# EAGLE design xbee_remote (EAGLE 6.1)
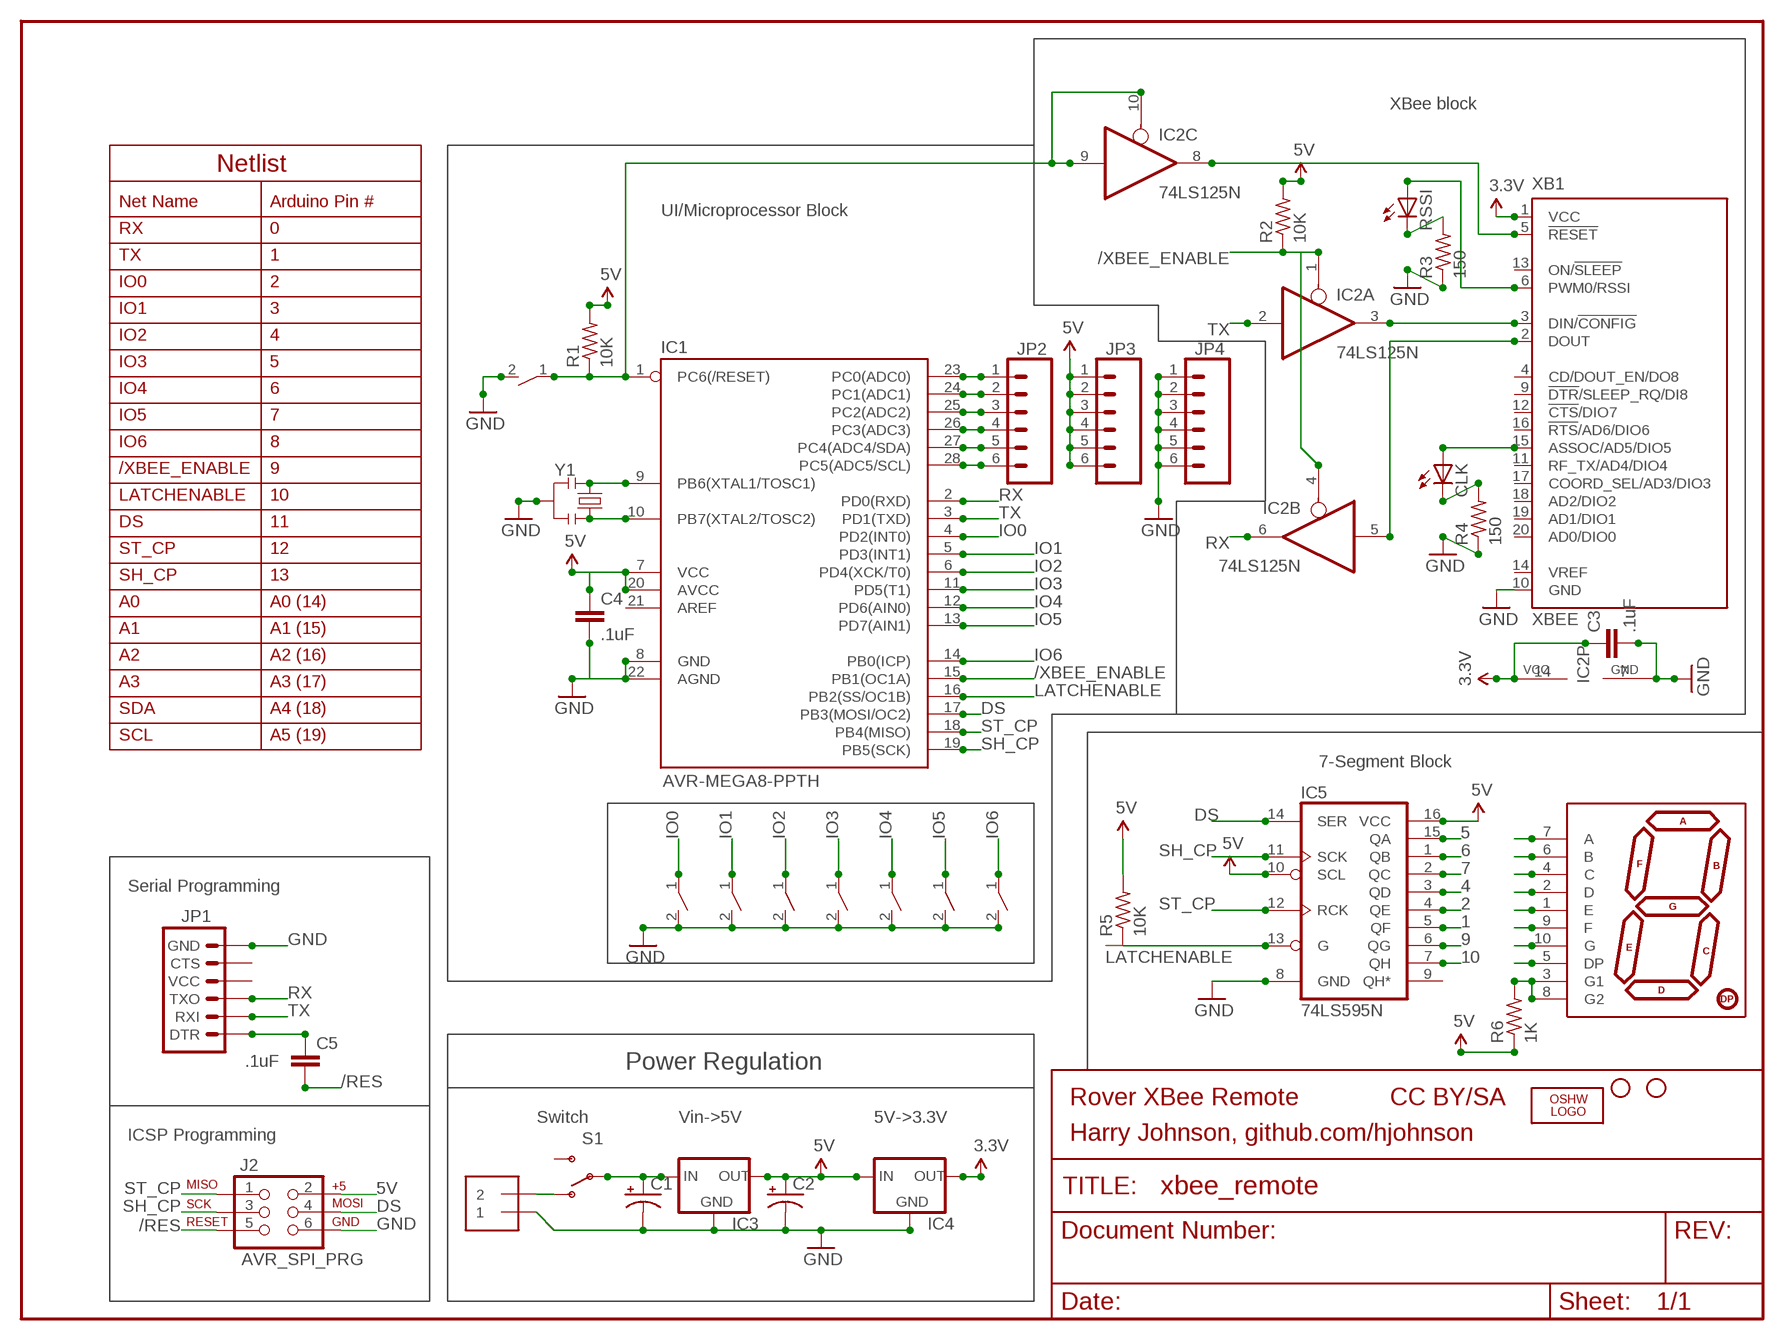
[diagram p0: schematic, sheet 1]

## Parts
C1  CAP_POLPTH1  [CPOL-RADIAL-100UF-25V]
C2  CAP_POLPTH2  [CPOL-RADIAL-10UF-25V]
C3  .1uF  CAPPTH2  [CAP-PTH-SMALL2]
C4  .1uF  CAPPTH2  [CAP-PTH-SMALL2]
C5  .1uF  CAPPTH2  [CAP-PTH-SMALL2]
CLK  LED3MM  [LED3MM]
IC1  AVR-MEGA8-PPTH  [DIL28-3]
IC2  74LS125N  [DIL14]
IC3  V_REG_78XXSIDE  [78XXL]
IC4  MCP1700TRI  [TO92]
IC5  74LS595N  [DIL16]
J1  1X2-3.5MM  [3.5MMTERM]
J2  AVR_SPI_PRG  AVR_SPI_PRG_6PTH  [2X3]
JP1  ARDUINO_SERIAL_PROGRAMPTH  [1X06]
JP2  M06SIP  [1X06]
JP3  M06SIP  [1X06]
JP4  M06SIP  [1X06]
JP5  STAND-OFF  [STAND-OFF]
JP6  STAND-OFF  [STAND-OFF]
LOGO1  OSHW_LOGO_FILLX0150-NT  [OSHW_FILLX150_NOTEXT]
R1  10K  R-US_0207/10  [0207/10]
R2  10K  R-US_0207/10  [0207/10]
R3  150  R-US_0207/10  [0207/10]
R4  150  R-US_0207/10  [0207/10]
R5  10K  R-US_0207/10  [0207/10]
R6  1K  R-US_0207/10  [0207/10]
RSSI  LED3MM  [LED3MM]
S1  SWITCH-SPSTPTH  [SWITCH-SPDT]
U$4  7-SEGMENT-DISPLAY-1"-RED  [7-SEGMENT-1"PTH]
U$8  TACT_TL1107  [TACT_TL1107]
U$9  TACT_TL1107  [TACT_TL1107]
U$10  TACT_TL1107  [TACT_TL1107]
U$11  TACT_TL1107  [TACT_TL1107]
U$12  TACT_TL1107  [TACT_TL1107]
U$13  TACT_TL1107  [TACT_TL1107]
U$14  TACT_TL1107  [TACT_TL1107]
U$15  TACT_TL1107  [TACT_TL1107]
XB1  XBEE  [XBEE]
Y1  RESONATORPTH  [RESONATOR-PTH]

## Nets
1: IC5.5(QF) U$4.1(E)
2: IC5.4(QE) U$4.2(D)
3.3V: C3.1 IC2.14(P:VCC) IC4.3(OUT) XB1.1(VCC)
3V3_/RST: IC2.8(C:O) XB1.5(!RESET)
3V3_RX: IC2.5(B:I) XB1.2(DOUT)
3V3_TX: IC2.3(A:O) XB1.3(DIN/!CONFIG)
4: IC5.3(QD) U$4.4(C)
5: IC5.15(QA) U$4.5(DP)
5V: C2.1(+) C4.1 IC1.7(VCC) IC1.20(AVCC) IC3.OUT IC4.2(IN) IC5.10(SCL) IC5.16(VCC) J2.2 JP3.1 JP3.2 JP3.3 JP3.4 JP3.5 JP3.6 R1.2 R2.2 R5.2 R6.1
6: IC5.1(QB) U$4.6(B)
7: IC5.2(QC) U$4.7(A)
9: IC5.6(QG) U$4.9(F)
10: IC5.7(QH) U$4.10(G)
/RES: C5.2 IC1.1(PC6(/RESET)) IC2.9(C:I) IC2.10(C:OE) J2.5 R1.1 U$8.1
/XBEE_ENABLE: IC1.15(PB1(OC1A)) IC2.1(A:OE) IC2.4(B:OE) R2.1
A0: IC1.23(PC0(ADC0)) JP2.1
A1: IC1.24(PC1(ADC1)) JP2.2
A2: IC1.25(PC2(ADC2)) JP2.3
A3: IC1.26(PC3(ADC3)) JP2.4
DS: IC1.17(PB3(MOSI/OC2)) IC5.14(SER) J2.4
GND: C1.2(-) C2.2(-) C3.2 C4.2 IC1.8(GND) IC1.22(AGND) IC2.7(P:GND) IC3.GND IC4.1(GND) IC5.8(GND) J1.1 J2.6 JP1.6(GND) JP4.1 JP4.2 JP4.3 JP4.4 JP4.5 JP4.6 R3.1 R4.1 U$8.2 U$9.2 U$10.2 U$11.2 U$12.2 U$13.2 U$14.2 U$15.2 XB1.10(GND) Y1.2
IO0: IC1.4(PD2(INT0)) U$9.1
IO1: IC1.5(PD3(INT1)) U$10.1
IO2: IC1.6(PD4(XCK/T0)) U$11.1
IO3: IC1.11(PD5(T1)) U$12.1
IO4: IC1.12(PD6(AIN0)) U$13.1
IO5: IC1.13(PD7(AIN1)) U$14.1
IO6: IC1.14(PB0(ICP)) U$15.1
LATCHENABLE: IC1.16(PB2(SS/OC1B)) IC5.13(G) R5.1
N$1: IC1.9(PB6(XTAL1/TOSC1)) Y1.1
N$2: IC1.10(PB7(XTAL2/TOSC2)) Y1.3
N$4: J1.2 S1.1(O)
N$5: C1.1(+) IC3.IN S1.2(P)
N$8: C5.1 JP1.1(DTR)
N$10: R6.2 U$4.3(G1) U$4.8(G2)
N$24: RSSI.A XB1.6(PWM0/RSSI)
N$25: R3.2 RSSI.K(C)
N$26: CLK.A XB1.15(ASSOC/AD5/DIO5)
N$27: CLK.K(C) R4.2
RX: IC1.2(PD0(RXD)) IC2.6(B:O) JP1.3(TXO)
SCL: IC1.28(PC5(ADC5/SCL)) JP2.6
SDA: IC1.27(PC4(ADC4/SDA)) JP2.5
SH_CP: IC1.19(PB5(SCK)) IC5.11(SCK) J2.3
ST_CP: IC1.18(PB4(MISO)) IC5.12(RCK) J2.1
TX: IC1.3(PD1(TXD)) IC2.2(A:I) JP1.2(RXI)
Unconnected: IC1.21(AREF) IC2.11(D:O) IC2.12(D:I) IC2.13(D:OE) IC5.9(QH*) JP1.4(VCC) JP1.5(CTS) S1.3(S) XB1.4(CD/DOUT_EN/DO8) XB1.9(!DTR!/SLEEP_RQ/DI8) XB1.11(RF_TX/AD4/DIO4) XB1.12(!CTS!/DIO7) XB1.13(ON/!SLEEP) XB1.14(VREF) XB1.16(!RTS!/AD6/DIO6) XB1.17(COORD_SEL/AD3/DIO3) XB1.18(AD2/DIO2) XB1.19(AD1/DIO1) XB1.20(AD0/DIO0)

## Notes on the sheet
- XBee block
- Netlist
- Net Name | Arduino Pin #
- UI/Microprocessor Block
- RX | 0
- TX | 1
- IO0 | 2
- IO1 | 3
- IO2 | 4
- IO3 | 5
- IO4 | 6
- IO5 | 7
- IO6 | 8
- /XBEE_ENABLE | 9
- LATCHENABLE | 10
- DS | 11
- ST_CP | 12
- SH_CP | 13
- A0 | A0 (14)
- A1 | A1 (15)
- A2 | A2 (16)
- A3 | A3 (17)
- SDA | A4 (18)
- SCL | A5 (19)
- 7-Segment Block
- Serial Programming
- Power Regulation
- Rover XBee Remote | CC BY/SA
- Switch | Vin->5V | 5V->3.3V
- ICSP Programming | Harry Johnson, github.com/hjohnson

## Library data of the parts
C1 C2 = SparkFun:CAP_POL: Capacitor Polarized
C3-C5 = SparkFun:CAP: Capacitor
CLK RSSI = adafruit:LED: LED
IC1 = SparkFun:AVR-MEGA8-P: MICROCONTROLLER 8 Kbytes FLASH 1 kbytes SRAM 512 bytes EEPROM USART 4-channel 10 bit ADC 2-channel 8 bit ADC
IC2 = 74xx-us:74*125: Quad bus BUFFER, 3-state
IC3 = SparkFun:V_REG_78XX: Voltage Regulator Standard 7805 5V regulator. IGO (Input Ground Output). Spark Fun Electronics SKU : COM-00107
IC4 = adafruit:MCP1700: VOLTAGE REGULATOR
IC5 = SparkFun:74*595: 8-bit SHIFT REGISTER, output latch
J1 = adafruit:1X2: 3.5mm Terminal block
J2 = SparkFun:AVR_SPI_PRG_6: AVR ISP 6 Pin This is the reduced ISP connector for AVR programming. Common on Arduino. This footprint will take up less PCB space and can be used with a 10-pin to 6-pin adapter such as SKU: BOB-08508
JP1 = SparkFun:ARDUINO_SERIAL_PROGRAM
JP2-JP4 = SparkFun:M06: Header 6 Standard 6-pin 0.1" header. Use with straight break away headers (SKU : PRT-00116), right angle break away headers (PRT-00553), swiss pins (PRT-00743), machine pins (PRT-00117), and female headers (PRT-00115). Molex polarized connector foot print use with SKU : PRT-08094 with associated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
JP5 JP6 = SparkFun:STAND-OFF: Stand Off
LOGO1 = OSHW:OSHW_LOGO_FILL
R1-R6 = adafruit:R-US_: RESISTOR, American symbol
S1 = SparkFun:SWITCH-SPST: SPST Switch Simple slide switch. Spark Fun Electronics SKU : COM-00102
U$4 = SparkFun:7-SEGMENT-DISPLAY-1"-RED: 7-Segment Display 1" Red (COM-08546)
U$8-U$15 = customswitch:TACT_TL1107: Tactile Switch, 2 pin, TL1107
XB1 = maxstream:XBEE: XBee (TM) /XBee-PRO(TM) OEM RF Modules Source: MaxStream, Inc. xbee_productmanual.pdf
Y1 = SparkFun:RESONATOR: Resonator Small SMD resonator. This is the itty bitty 10/20MHz resonators with built in caps. CSTCE10M0G55 and CSTCE20M0V53. Footprint has been reviewed closely but hasn't been tested yet.

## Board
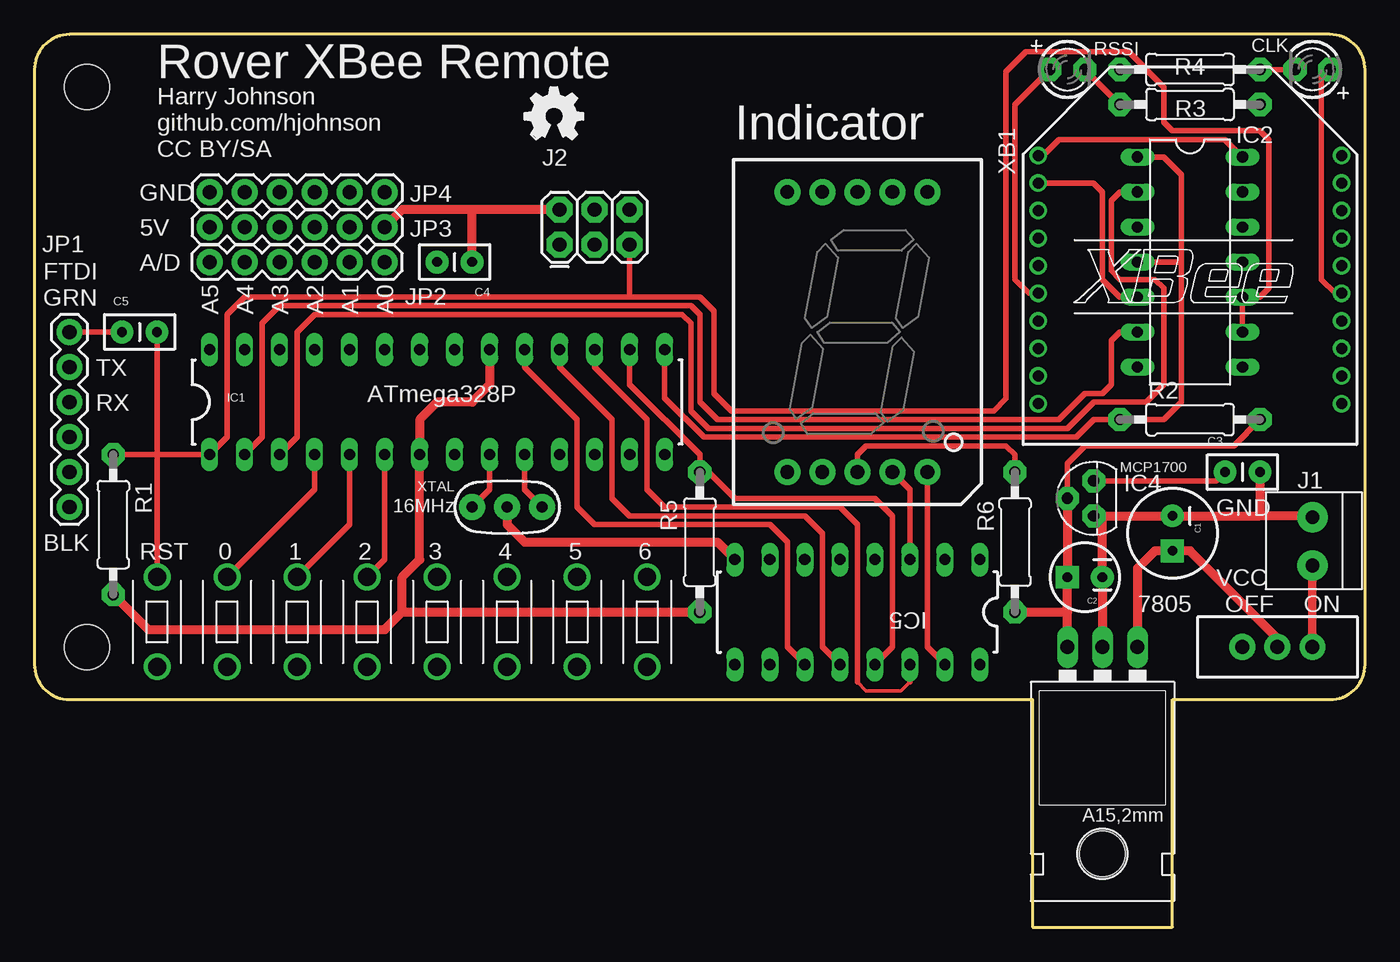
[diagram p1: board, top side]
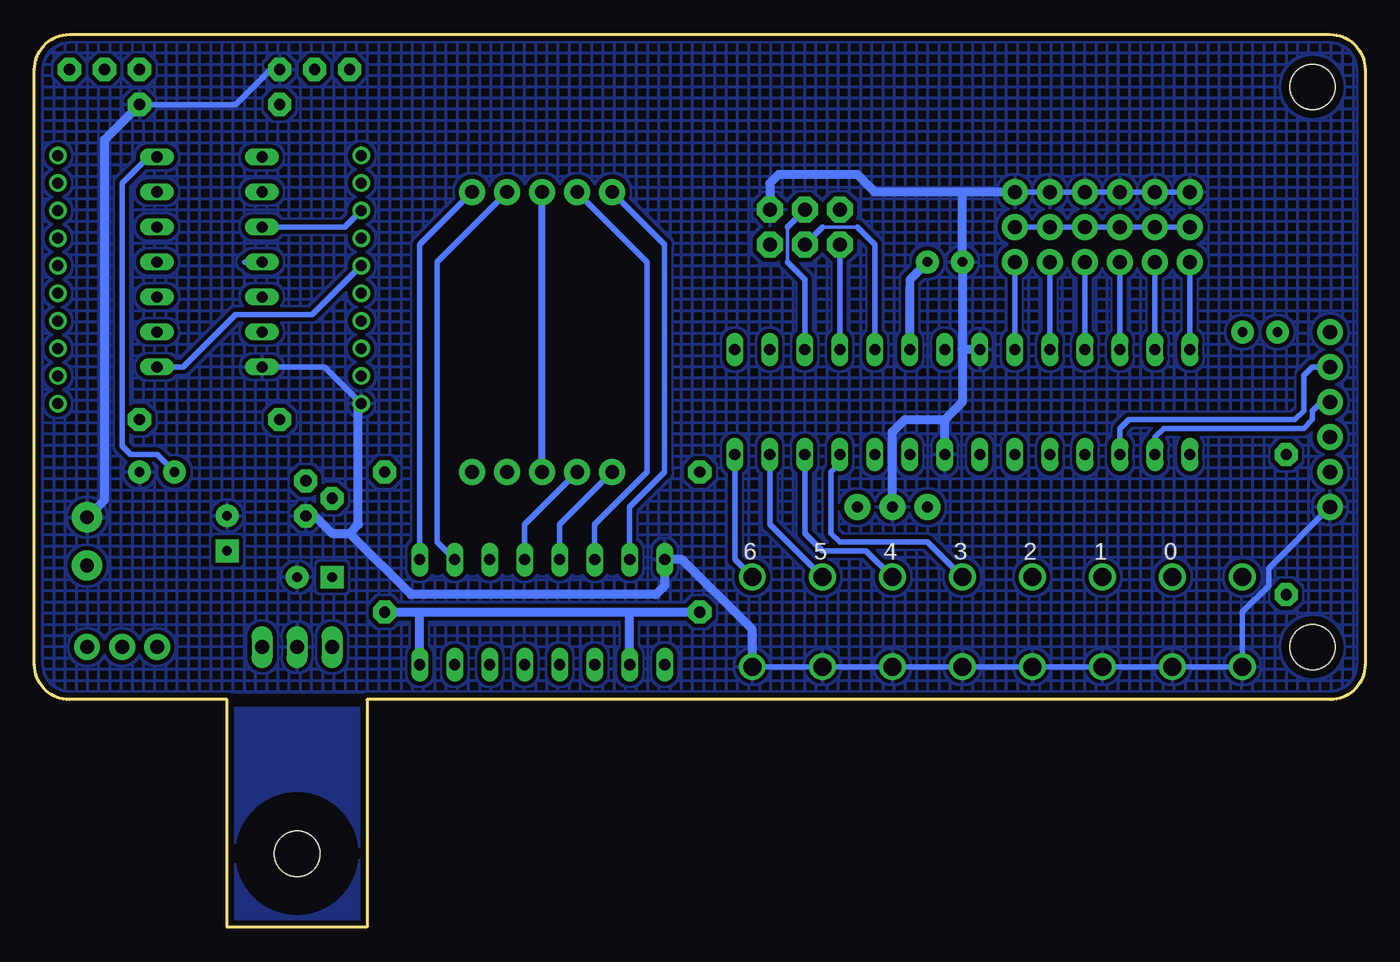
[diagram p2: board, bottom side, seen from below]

Size 96.52 x 64.77 mm. Coordinates in mm from the lower left corner, seen from the top.
Outline: 0,19.05 arc90 2.54,16.51 72.39,16.51 72.39,0 82.55,0 82.55,16.51 93.98,16.51 arc90 96.52,19.05 96.52,62.23 arc90 93.98,64.77 2.54,64.77 arc90 0,62.23 0,19.05
Copper layers (1*16): Top 0.0356mm / dielectric 1.5011mm / Bottom 0.0356mm
Design rules: minimum track width 6mil, minimum drill 13mil, track to track 6mil, track to pad 6mil, pad to pad 6mil, via to via 6mil, smd to smd 6mil, copper to edge 15mil, drill to drill 6mil, minimum pad ring 7mil, minimum via ring 7mil, stop-mask expansion 4mil, vias tented up to drill 0mil, thermal gap 10mil
tRestrict: 1 lines
bRestrict: 7 lines

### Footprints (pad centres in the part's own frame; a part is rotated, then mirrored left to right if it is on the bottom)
CPOL-RADIAL-100UF-25V = drill 0.7 pad 1.651 square: 1 1.27,0 | drill 0.7 pad 1.651: 2 -1.27,0
CPOL-RADIAL-10UF-25V = drill 0.7 pad 1.651 square: 1 1.27,0 | drill 0.7 pad 1.651: 2 -1.27,0
CAP-PTH-SMALL2 = drill 0.7 pad 1.651: 1 0,0; 2 2.54,0
LED3MM = drill 0.813 pad 1.676 octagon: A -1.27,0; K 1.27,0
DIL28-3 = drill 0.813 long: 1 -16.51,-3.81; 2 -13.97,-3.81; 3 -11.43,-3.81; 4 -8.89,-3.81; 5 -6.35,-3.81; 6 -3.81,-3.81; 7 -1.27,-3.81; 8 1.27,-3.81; 9 3.81,-3.81; 10 6.35,-3.81; 11 8.89,-3.81; 12 11.43,-3.81; 13 13.97,-3.81; 14 16.51,-3.81; 15 16.51,3.81; 16 13.97,3.81; 17 11.43,3.81; 18 8.89,3.81; 19 6.35,3.81; 20 3.81,3.81; 21 1.27,3.81; 22 -1.27,3.81; 23 -3.81,3.81; 24 -6.35,3.81; 25 -8.89,3.81; 26 -11.43,3.81; 27 -13.97,3.81; 28 -16.51,3.81
DIL14 = drill 0.813 long: 1 -7.62,-3.81; 2 -5.08,-3.81; 3 -2.54,-3.81; 4 0,-3.81; 5 2.54,-3.81; 6 5.08,-3.81; 7 7.62,-3.81; 8 7.62,3.81; 9 5.08,3.81; 10 2.54,3.81; 11 0,3.81; 12 -2.54,3.81; 13 -5.08,3.81; 14 -7.62,3.81
78XXL = drill 1.016 long: GND 0,-3.81; IN -2.54,-3.81; OUT 2.54,-3.81 | hole 3.302: 0,11.176
TO92 = drill 0.813 pad 1.676 octagon: 1 -1.27,0; 2 0,1.905; 3 1.27,0
DIL16 = drill 0.813 long: 1 -8.89,-3.81; 2 -6.35,-3.81; 3 -3.81,-3.81; 4 -1.27,-3.81; 5 1.27,-3.81; 6 3.81,-3.81; 7 6.35,-3.81; 8 8.89,-3.81; 9 8.89,3.81; 10 6.35,3.81; 11 3.81,3.81; 12 1.27,3.81; 13 -1.27,3.81; 14 -3.81,3.81; 15 -6.35,3.81; 16 -8.89,3.81
3.5MMTERM = drill 1 pad 2.184: 1 1.8,0; 2 -1.7,0
2X3 = drill 1.016 pad 1.88 octagon: 1 0,0; 2 0,2.54; 3 2.54,0; 4 2.54,2.54; 5 5.08,0; 6 5.08,2.54
1X06 = drill 1.016 pad 1.88: 1 0,0; 2 2.54,0; 3 5.08,0; 4 7.62,0; 5 10.16,0; 6 12.7,0
STAND-OFF = hole 3.302: 0,0
0207/10 = drill 0.813 pad 1.676 octagon: 1 -5.08,0; 2 5.08,0
SWITCH-SPDT = drill 1.016 pad 1.88: 1 0,2.54; 2 0,0; 3 0,-2.54
7-SEGMENT-1"PTH = drill 1 pad 1.88: 1 -5.08,-10.16; 2 -2.54,-10.16; 3 0,-10.16; 4 2.54,-10.16; 5 5.08,-10.16; 6 5.08,10.16; 7 2.54,10.16; 8 0,10.16; 9 -2.54,10.16; 10 -5.08,10.16
TACT_TL1107 = drill 1.3: 1 0,0; 2 6.5,0
XBEE = drill 0.8 pad 1.27: 1 -11,9; 2 -11,7; 3 -11,5; 4 -11,3; 5 -11,1; 6 -11,-1; 7 -11,-3; 8 -11,-5; 9 -11,-7; 10 -11,-9; 11 11,-9; 12 11,-7; 13 11,-5; 14 11,-3; 15 11,-1; 16 11,1; 17 11,3; 18 11,5; 19 11,7; 20 11,9
RESONATOR-PTH = drill 0.8 pad 1.88: 1 -2.54,0; 2 0,0; 3 2.54,0

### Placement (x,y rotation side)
C1  82.55,28.57 270 top
C2  76.2,25.4 180 top
C3  86.36,33.02 0 top
C4  31.75,48.26 180 top
C5  6.35,43.18 0 top
CLK  92.71,62.23 180 top
IC1  29.21,38.1 0 top
IC2  83.82,48.26 270 top
IC3  77.47,16.51 180 top
IC4  76.83,31.11 90 top
IC5  59.69,22.86 180 top
J1  92.71,27.94 90 top
J2  38.1,49.53 0 top
JP1  2.54,43.18 270 top
JP2  25.4,48.26 180 top
JP3  12.7,50.8 0 top
JP4  12.7,53.34 0 top
JP5  3.81,20.32 0 top
JP6  3.81,60.96 0 top
LOGO1  35.56,57.15 0 top
R1  5.71,29.21 270 top
R2  83.82,36.83 0 top
R3  83.82,59.69 180 top
R4  83.82,62.23 0 top
R5  48.26,27.94 270 top
R6  71.12,27.94 90 top
RSSI  74.93,62.23 0 top
S1  90.17,20.32 270 top
U$4  59.69,43.18 0 top
U$8  8.89,25.4 270 top
U$9  13.97,25.4 270 top
U$10  19.05,25.4 270 top
U$11  24.13,25.4 270 top
U$12  29.21,25.4 270 top
U$13  34.29,25.4 270 top
U$14  39.37,25.4 270 top
U$15  44.45,25.4 270 top
XB1  83.82,46.99 0 top
Y1  34.29,30.48 0 top

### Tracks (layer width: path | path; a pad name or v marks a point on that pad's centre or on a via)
1
  Bottom 0.406: IC5.5 58.42,29.21 U$4.1
2
  Bottom 0.406: IC5.4 60.96,29.21 U$4.2
3.3V
  Top 0.406: IC2.14 86.36,57.15 74.3,57.15 73.14,55.99 XB1.1 | IC4.3 85.72,32.38 C3.1
  Bottom 0.406: IC2.14 88.27,55.88 90.17,53.98 90.17,34.92 89.53,34.29 87.63,34.29 C3.1
3V3_/RST
  Bottom 0.406: IC2.8 85.72,40.64 81.92,44.45 76.36,44.45 XB1.5
3V3_RX
  Top 0.406: IC2.5 78.74,45.72 77.47,46.99 77.47,53.34 76.82,53.99 XB1.2
3V3_TX
  Bottom 0.406: IC2.3 74.01,50.8 XB1.3
4
  Top 0.406: IC5.3 63.5,31.75 U$4.4
5
  Top 0.406: IC5.15 64.77,20.32 U$4.5
5V
  Top 0.406: IC4.2 74.93,33.66 76.2,34.92 87,34.92 R2.2
  Top 0.635: R1.2 8.26,21.59 25.4,21.59 26.67,22.86 | 26.67,22.86 26.67,25.4 27.94,26.67 IC1.7 27.94,36.83 29.21,38.1 31.75,38.1 33.02,39.37 IC1.20 | 26.67,22.86 R5.2 | IC3.OUT 74.93,22.86 | 74.93,22.86 C2.1 IC4.2 | R6.1 74.93,22.86 | J2.2 31.75,52.07 | 31.75,52.07 26.67,52.07 JP3.6 | C4.1 31.75,52.07
  Bottom 0.406: JP3.6 JP3.5 JP3.4 JP3.3 JP3.2 JP3.1
  Bottom 0.61: 33.02,46.35 33.02,46.99 C4.1
  Bottom 0.635: IC1.20 33.02,46.35 | R6.1 68.58,22.86 | 68.58,22.86 53.34,22.86 | 53.34,22.86 R5.2 | IC5.10 53.34,22.86 | IC5.16 68.58,22.86
6
  Bottom 0.406: IC5.1 68.58,49.53 U$4.6
7
  Bottom 0.406: IC5.2 67.31,27.94 67.31,48.26 U$4.7
9
  Bottom 0.406: U$4.9 52.07,48.26 52.07,33.02 55.88,29.21 IC5.6
10
  Bottom 0.406: U$4.10 50.8,49.53 50.8,33.02 53.34,30.48 IC5.7
/RES
  Top 0.406: 8.89,34.29 C5.2 | IC2.9 IC2.10 88.9,45.72 89.53,46.35 89.53,57.15 88.9,57.78 82.55,57.78 81.92,58.42 81.92,60.96 79.38,63.5 71.91,63.5 70.48,62.08 70.48,38.36 69.59,37.47 50.55,37.47 49.28,38.73 49.28,44.7 48.26,45.72 43.18,45.72 | 8.89,34.29 R1.1 | 8.89,34.29 IC1.1 13.97,35.56 13.97,44.45 15.24,45.72 43.18,45.72 | U$8.1 8.89,34.29 | 43.18,45.72 J2.5
/XBEE_ENABLE
  Top 0.406: 83.19,48.26 83.19,38.1 81.92,36.83 R2.1 76.83,36.83 75.56,35.56 48.56,35.56 45.72,38.4 IC1.15 | 83.19,48.26 IC2.4 | IC2.1 81.92,55.88 83.19,54.61 83.19,48.26
  Bottom 0.406: IC2.4 81.28,48.26
A0
  Bottom 0.406: IC1.23 JP2.1
A1
  Bottom 0.406: IC1.24 JP2.2
A2
  Bottom 0.406: IC1.25 JP2.3
A3
  Bottom 0.406: IC1.26 JP2.4
DS
  Top 0.254: 59.69,17.78 60.33,17.14 62.87,17.14 63.5,17.78
  Top 0.406: 59.69,17.78 59.69,29.21 58.42,30.48 45.72,30.48 44.45,31.75 44.45,36.83 40.64,40.64 IC1.17 | 63.5,17.78 IC5.14
  Bottom 0.254: 41.91,48.26 41.91,50.8
  Bottom 0.406: 41.91,50.8 J2.4 | 41.91,48.26 40.64,46.99 IC1.17
GND
  Top 0.635: 77.47,29.84 C2.2 IC3.GND | 88.9,29.84 C1.2 77.47,29.84 | IC4.1 77.47,29.84 | C3.2 88.9,29.84 | Y1.2 34.29,29.21 35.56,27.94 49.53,27.94 IC5.8 | 88.9,29.84 92.61,29.84 J1.1
  Bottom 0.406: U$15.2 U$14.2 U$13.2 U$12.2 U$11.2 U$10.2 U$9.2 U$8.2 8.89,22.86 6.99,24.77 6.99,26.04 JP1.6 | XB1.10 75.47,40.64 IC2.7 | R4.1 79.38,62.23 81.92,59.69 R3.1 | JP4.1 JP4.2 JP4.3 JP4.4 JP4.5 JP4.6
  Bottom 0.635: IC1.8 30.48,36.83 | JP4.6 29.21,53.34 | 29.21,53.34 35.56,53.34 36.83,54.61 42.55,54.61 43.18,53.98 J2.6 | Y1.2 34.29,35.93 33.39,36.83 30.48,36.83 | 29.21,41.91 C4.2 29.21,53.34 | 29.21,41.91 29.21,38.1 30.48,36.83 | IC1.22 29.21,41.91 | 72.71,38.1 XB1.10 73.03,37.78 73.03,29.21 73.66,28.57 | IC4.1 76.2,29.84 74.93,28.57 73.66,28.57 | U$15.2 44.45,21.59 49.53,26.67 IC5.8 50.8,24.77 51.44,24.13 69.22,24.13 73.66,28.57 | J1.1 91.44,31.01 91.44,57.15 R3.1
  pour Bottom (isolate 0.305, hatched): 0,16.51 96.52,16.51 96.52,64.77 0,64.77
IO0
  Top 0.406: U$9.1 20.32,31.75 IC1.4
IO1
  Top 0.406: U$10.1 22.86,29.21 IC1.5
IO2
  Top 0.406: U$11.1 25.4,26.67 IC1.6
IO3
  Bottom 0.406: U$12.1 31.75,27.94 38.1,27.94 38.73,28.57 38.73,33.02 38.1,33.66 IC1.11
IO4
  Bottom 0.406: U$13.1 36.2,27.3 39.37,27.3 40.64,28.57 IC1.12
IO5
  Bottom 0.406: U$14.1 43.18,29.21 IC1.13
IO6
  Bottom 0.406: U$15.1 45.72,26.67 IC1.14
LATCHENABLE
  Top 0.406: IC5.13 62.23,20.32 62.23,29.84 60.96,31.11 50.8,31.11 48.9,33.02 R5.1 48.26,34.29 43.18,39.37 IC1.16
N$1
  Top 0.406: Y1.1 33.02,31.75 IC1.9
N$2
  Top 0.406: Y1.3 35.56,31.75 IC1.10
N$3
  pour Bottom (isolate 0.254, no thermals): 72.39,15.88 82.55,15.88 82.55,0 72.39,0
N$4
  Top 0.61: J1.2 S1.1
N$5
  Top 0.61: 87.63,23.5 90.17,20.95 S1.2
  Top 0.635: 87.63,23.5 83.82,27.3 C1.1 81.28,27.3 80.01,26.04 IC3.IN
N$8
  Top 0.406: JP1.1 C5.1
N$10
  Top 0.406: R6.2 71.12,34.29 70.48,34.92 60.33,34.92 59.69,34.29 U$4.3
  Bottom 0.508: U$4.3 U$4.8
N$24
  Top 0.406: RSSI.A 71.12,59.69 71.12,46.99 72.12,45.99 XB1.6
N$25
  Top 0.406: R3.2 RSSI.K
N$26
  Top 0.406: XB1.15 94.34,45.99 93.34,46.99 93.34,61.59 CLK.A
N$27
  Top 0.406: R4.2 CLK.K
RX
  Top 0.406: IC2.6 78.74,43.18 78.11,42.55 78.11,39.37 77.47,38.73 76.2,38.73 74.3,36.83 49.53,36.83 48.26,38.1 48.26,44.45 47.62,45.09 17.78,45.09 16.51,43.81 16.51,35.56 IC1.2
  Bottom 0.406: IC1.2 15.24,35.56 14.61,36.2 4.45,36.2 3.81,36.83 3.81,37.47 3.17,38.1 JP1.3
SCL
  Bottom 0.406: IC1.28 JP2.6
SDA
  Bottom 0.406: IC1.27 JP2.5
SH_CP
  Top 0.406: IC5.11 54.61,20.32 54.61,27.94 53.34,29.21 40.64,29.21 39.37,30.48 39.37,36.83 35.56,40.64 IC1.19
  Bottom 0.254: 36.83,50.8 39.37,50.8
  Bottom 0.406: 39.37,50.8 J2.3 | 36.83,50.8 35.56,49.53 IC1.19
ST_CP
  Top 0.406: IC5.12 57.15,20.32 57.15,28.57 55.88,29.84 43.18,29.84 41.91,31.11 41.91,36.83 38.1,40.64 IC1.18
  Bottom 0.406: IC1.18 J2.1
TX
  Top 0.406: IC2.2 78.74,53.34 78.11,52.7 78.11,47.62 78.74,46.99 81.28,46.99 81.92,46.35 81.92,39.37 80.64,38.1 76.83,38.1 74.93,36.2 48.9,36.2 47.62,37.47 47.62,43.81 46.99,44.45 20.32,44.45 19.05,43.18 19.05,35.56 IC1.3
  Bottom 0.406: IC1.3 17.78,36.2 17.14,36.83 5.08,36.83 4.45,37.47 4.45,40.01 3.81,40.64 JP1.2

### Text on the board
tPlace: Rover XBee Remote | Harry Johnson | github.com/hjohnson | Indicator | CC BY/SA | GND | 5V | A/D | FTDI | GRN | A5 | A4 | A3 | A2 | A1 | A0 | TX | ATmega328P | RX | MCP1700 | XTAL | 16MHz | GND | BLK | RST | 0 | 1 | 2 | 3 | 4 | 5 | 6 | VCC | 7805 | OFF | ON
bPlace: 0 | 1 | 2 | 3 | 4 | 5 | 6
Reference: 7-Segment block | XBEE block | Prog Block | VREG Block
